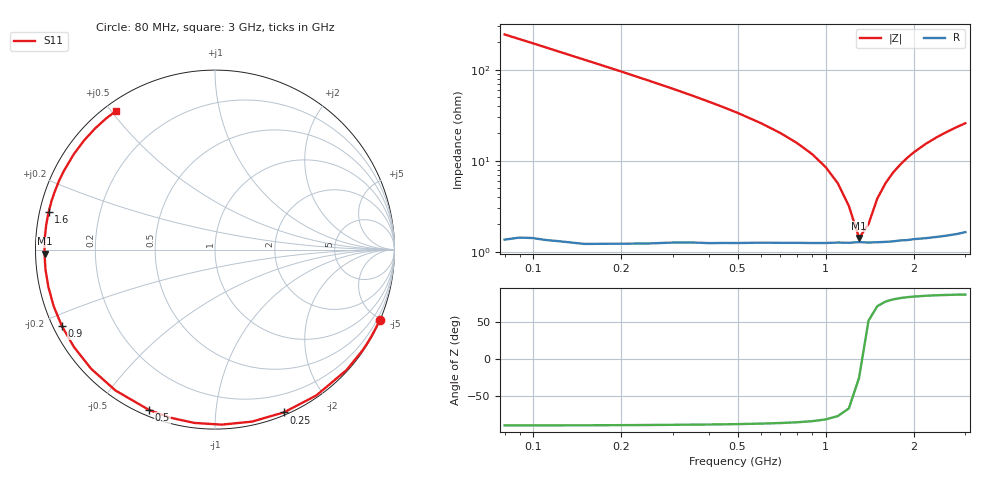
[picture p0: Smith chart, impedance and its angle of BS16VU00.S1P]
! SIEMENS Small Signal Semiconductors
! BB640
! Si Tuning Diode in SOD323
! VR = 16 V
! S-Parameters:  July  1993
# GHz  S  MA  R  50
!  f  S11
! GHz  MAG  ANG
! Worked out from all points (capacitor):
!   33 points, 80 MHz to 3 GHz, reference 50 ohm
!   read as one part to ground: C = 8.13 pF near 80 MHz
!   lowest |Z| = 1.42 ohm at 1.3 GHz (marker M1)
!   series resonance near 1.328 GHz, so ESL is about 1.8 nH
!   S11 on the Smith chart (normalised r, x): 80 MHz: 0.03, -4.87; 250 MHz: 0.02, -1.51; 500 MHz: 0.02, -0.67; 900 MHz: 0.03, -0.23; 1.6 GHz: 0.03, +0.11; 3 GHz: 0.03, +0.52
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0.08  0.9978 -23.2
0.1  0.9965 -28.8
0.12  0.9954 -34.4
0.15  0.9936 -42.5
0.2  0.9895 -55.2
0.25  0.985 -67.1
0.3  0.9802 -77.9
0.35  0.9759 -87.8
0.4  0.9725 -96.8
0.45  0.969 -104.9
0.5  0.9661 -112.3
0.6  0.961 -125.2
0.7  0.9577 -136.1
0.8  0.9552 -145.5
0.9  0.9537 -153.6
1  0.9525 -160.9
1.1  0.9512 -167.4
1.2  0.9511 -173.3
1.3  0.9501 -178.6
1.5  0.9505 171.7
1.6  0.9504 167.4
1.8  0.9496 159.5
2  0.9493 152.3
2.2  0.9496 145.9
2.4  0.9497 140.1
2.6  0.9498 134.8
2.8  0.9498 129.9
3  0.9493 125.4
